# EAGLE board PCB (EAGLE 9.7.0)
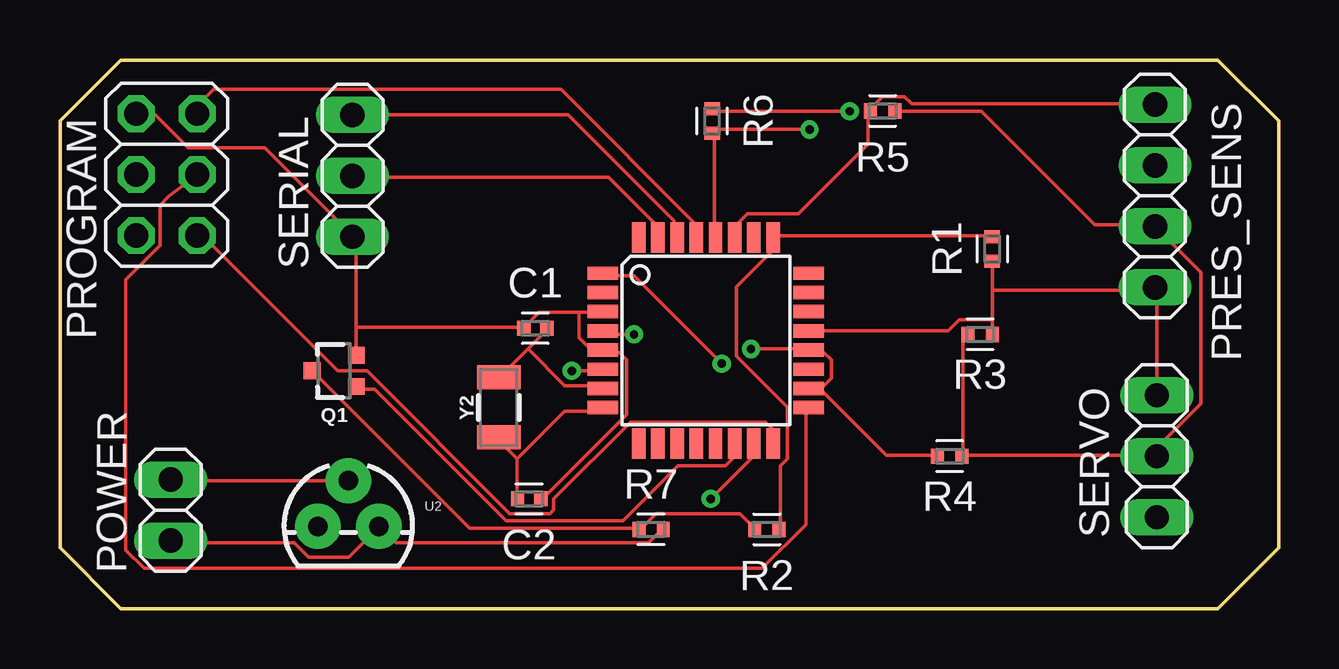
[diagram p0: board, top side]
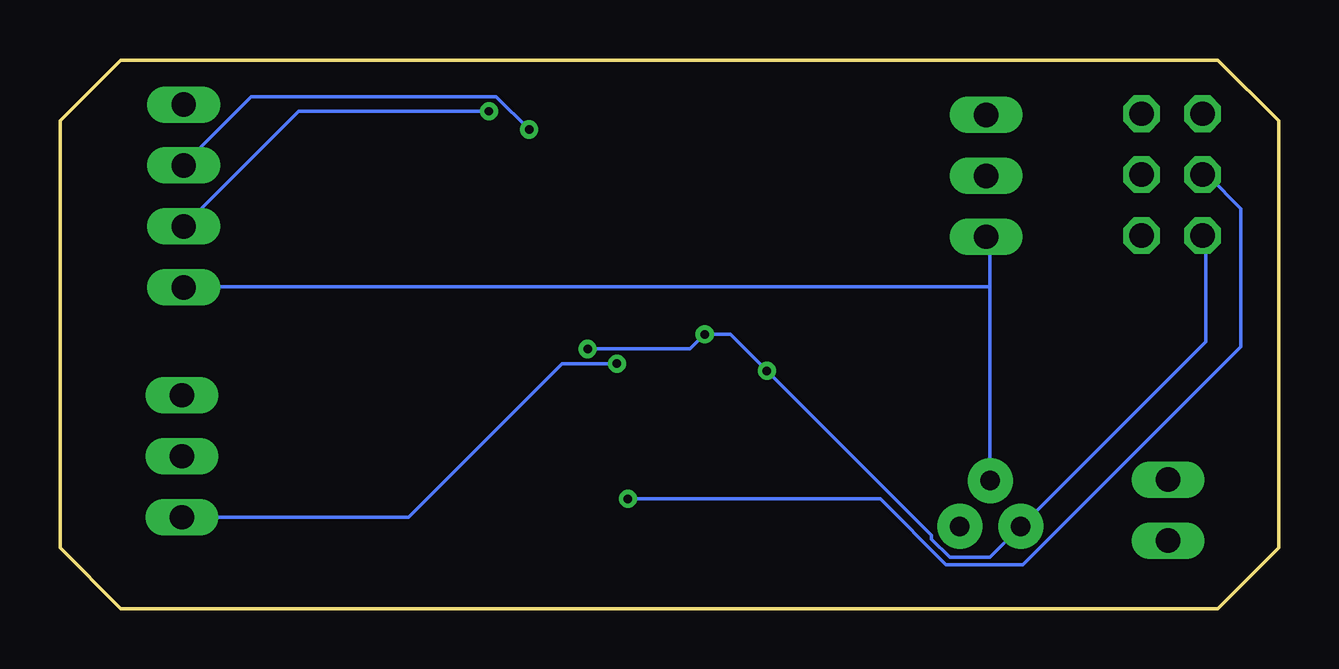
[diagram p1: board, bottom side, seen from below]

Size 50.8 x 22.86 mm. Coordinates in mm from the lower left corner, seen from the top.
Outline: 0,2.54 0,20.32 2.54,22.86 48.26,22.86 50.8,20.32 50.8,2.54 48.26,0 2.54,0 0,2.54
Copper layers (1*16): Top 0.035mm / dielectric 1.5mm / Bottom 0.035mm
Design rules "default": minimum track width 6mil, minimum drill 0.35mm, track to track 6mil, track to pad 6mil, pad to pad 6mil, via to via 6mil, smd to smd 6mil, copper to edge 40mil, drill to drill 6mil, minimum pad ring 10mil, minimum via ring 8mil, stop-mask expansion 4mil, vias tented up to drill 0mil, thermal gap 10mil

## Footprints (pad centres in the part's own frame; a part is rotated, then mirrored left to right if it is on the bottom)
CAPC1005X60 = smd 0.56 x 0.629: 1 -0.485,0; 2 0.485,0
TQFP32-08 = smd 1.27 x 0.559: 1 -4.293,2.8; 2 -4.293,2; 3 -4.293,1.2; 4 -4.293,0.4; 5 -4.293,-0.4; 6 -4.293,-1.2; 7 -4.293,-2; 8 -4.293,-2.8; 17 4.293,-2.8; 18 4.293,-2; 19 4.293,-1.2; 20 4.293,-0.4; 21 4.293,0.4; 22 4.293,1.2; 23 4.293,2; 24 4.293,2.8 | smd 0.559 x 1.27: 9 -2.8,-4.293; 10 -2,-4.293; 11 -1.2,-4.293; 12 -0.4,-4.293; 13 0.4,-4.293; 14 1.2,-4.293; 15 2,-4.293; 16 2.8,-4.293; 25 2.8,4.293; 26 2,4.293; 27 1.2,4.293; 28 0.4,4.293; 29 -0.4,4.293; 30 -1.2,4.293; 31 -2,4.293; 32 -2.8,4.293
1X02 = drill 1.016 long: 1 -1.27,0; 2 1.27,0
1X04 = drill 1.016 long: 1 -3.81,0; 2 -1.27,0; 3 1.27,0; 4 3.81,0
2X03 = drill 1.016 octagon: 1 -2.54,-1.27; 2 -2.54,1.27; 3 0,-1.27; 4 0,1.27; 5 2.54,-1.27; 6 2.54,1.27
SOT323 = smd 0.7 x 0.7: 1 -0.65,-0.925; 2 0.65,-0.925; 3 0,0.925
RESC1005X40 = smd 0.535 x 0.644: 1 -0.507,0; 2 0.507,0
1X03 = drill 1.016 long: 1 -2.54,0; 2 0,0; 3 2.54,0
TO-92 = drill 0.813 pad 1.88: 1 -1.27,0; 2 0,1.905; 3 1.27,0
CRYSTAL-SMD-3.2X1.5MM = smd 1 x 1.8: P$1 -1.25,0; P$2 1.25,0

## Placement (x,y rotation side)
C1  22p  [CAPC1005X60]  19.81,11.68 0 top
C2  22p  [CAPC1005X60]  19.56,4.57 180 top
IC1  ATMEGA328P  [TQFP32-08]  26.92,11.18 0 top
POWER  PINHD-1X2  [1X02]  4.61,4.11 90 top
PRES_SENS  PINHD-1X4  [1X04]  45.64,17.2 270 top
PROGRAM  PINHD-2X3  [2X03]  4.45,18.08 90 top
Q1  310mA/60V/1.6Ω  [SOT323]  11.43,9.91 90 top
R1  10K  [RESC1005X40]  38.86,14.99 90 top
R2  5K  [RESC1005X40]  29.46,3.3 180 top
R3  5K  [RESC1005X40]  38.35,11.43 0 top
R4  5K  [RESC1005X40]  37.08,6.35 0 top
R5  5K  [RESC1005X40]  34.29,20.74 180 top
R6  5K  [RESC1005X40]  27.18,20.32 270 top
R7  10K  [RESC1005X40]  24.64,3.3 0 top
SERIAL  PINHD-1X3  [1X03]  12.19,18.03 90 top
SERVO  PINHD-1X3  [1X03]  45.72,6.35 270 top
U2  7805  [TO-92]  12.02,3.43 0 top
Y2  16M  [CRYSTAL-SMD-3.2X1.5MM]  18.29,8.38 90 top

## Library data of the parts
C1 C2 = Capacitor; CATEGORY: Capacitor
IC1 = IC_Embedded; CATEGORY: IC_Embedded; MANUFACTURER: Microchip; MPN: ATmega328P-MMH; OPERATING_TEMP: -40 to 85 °C; PART_STATUS: Active; SUB-CATEGORY: Microcontroller
POWER PRES_SENS PROGRAM SERIAL SERVO = Connector; CATEGORY: CONNECTOR; SUB-CATEGORY: PIN-HEADER
Q1 = SparkFun-DiscreteSemi; PROD_ID: TRANS-11151
R1-R7 = Resistor; CATEGORY: Resistor; SUB-CATEGORY: Fixed
U2 = SparkFun-IC-Power
Y2 = SparkFun-Clocks

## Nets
+V: POWER.1 R7.2 U2.3
GND: C1.1 C2.1 IC1.3 IC1.5 IC1.21 POWER.2 PRES_SENS.4 PROGRAM.6 Q1.2 R1.1 R3.2 SERIAL.1 SERVO.1 U2.2
N$1: IC1.4 IC1.6 IC1.18 IC1.20 PROGRAM.2 R4.1 U2.1
N$2: C1.2 IC1.7 Y2.P$2
N$3: C2.2 IC1.8 Y2.P$1
N$4: IC1.28 PRES_SENS.2 R6.2
N$5: IC1.27 PRES_SENS.1 R5.2
N$7: IC1.14 Q1.1
N$8: IC1.25 R1.2 R2.1
N$9: Q1.3 R2.2 R7.1
N$10: PRES_SENS.3 R3.1 R4.2 R5.1 R6.1 SERVO.2
N$11: IC1.16 PROGRAM.1
N$12: IC1.17 PROGRAM.3
N$13: IC1.29 PROGRAM.5
N$14: IC1.15 PROGRAM.4
N$17: IC1.1 SERVO.3
N$18: IC1.31 SERIAL.2
N$19: IC1.30 SERIAL.3

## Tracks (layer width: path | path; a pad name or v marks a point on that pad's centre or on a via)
+V
  Top 0.152: R7.2 24.99,3.2 24.54,2.74 14.02,2.74 13.41,3.35 U2.3 13.26,3.35 12.04,2.13 10.36,2.13 9.75,2.74 4.72,2.74 POWER.1
GND
  Top 0.152: R1.1 38.86,13.26 | 38.86,13.26 38.86,12.04 | 38.86,12.04 R3.2 | 38.86,12.04 37.49,12.04 37.03,11.58 31.24,11.58 IC1.21 | SERVO.1 45.72,13.26 PRES_SENS.4 45.57,13.26 38.86,13.26 | U2.2 4.72,5.33 POWER.2 | 21.64,12.34 22.55,12.34 IC1.3 | 21.64,12.34 19.96,12.34 19.36,11.73 C1.1 19.2,11.73 12.34,11.73 | C2.1 20.12,4.57 23.62,8.08 23.62,10.36 23.32,10.67 22.71,10.67 IC1.5 22.55,10.82 22.1,10.82 21.64,11.28 21.64,12.34 | 12.34,11.73 12.34,15.24 12.19,15.39 SERIAL.1 12.19,15.54 8.53,19.2 5.33,19.2 3.96,20.57 3.3,20.57 PROGRAM.6 | 12.34,11.73 12.34,10.67 Q1.2
  Bottom 0.152: 12.04,13.41 12.04,15.24 12.19,15.39 SERIAL.1 | 12.04,13.41 12.04,5.33 U2.2 | 12.04,13.41 45.57,13.41 PRES_SENS.4
N$1  (via drill 0.35)
  Top 0.152: 31.7,9.14 34.44,6.4 36.58,6.4 R4.1 | 31.7,9.14 31.24,9.14 IC1.18 31.7,9.14 | 31.7,9.14 32.16,9.6 32.16,10.36 31.85,10.67 31.24,10.67 IC1.20 31.09,10.82 v28.8,10.82 | v21.34,9.91 22.55,9.91 IC1.6 | v23.93,11.43 22.71,11.43 IC1.4
  Bottom 0.152: PROGRAM.2 3.05,15.38 3.05,11.12 10.67,3.5 U2.1 10.82,3.35 12.04,2.13 13.72,2.13 14.48,2.9 14.48,3.05 v21.34,9.91 22.86,11.43 v23.93,11.43 24.54,10.82 v28.8,10.82
N$2
  Top 0.152: 19.51,10.82 18.29,9.6 Y2.P$2 | 19.51,10.82 20.27,11.58 C1.2 | 19.51,10.82 21.03,9.3 22.55,9.3 IC1.7
N$3
  Top 0.152: 19.05,6.25 19.05,4.57 C2.2 | 19.05,6.25 18.29,7.01 Y2.P$1 | 19.05,6.25 21.03,8.23 22.55,8.23 IC1.8
N$4  (via drill 0.35)
  Top 0.152: IC1.28 27.28,15.54 27.28,19.81 R6.2 27.28,19.96 v31.24,19.96
  Bottom 0.152: v31.24,19.96 32.61,21.34 42.82,21.34 45.57,18.59 PRES_SENS.2
N$5
  Top 0.152: IC1.27 28.19,15.54 28.19,16 28.65,16.46 30.79,16.46 33.68,19.36 33.68,20.73 R5.2 33.83,20.88 34.29,21.34 35.2,21.34 35.51,21.03 45.57,21.03 PRES_SENS.1
N$7
  Top 0.152: Q1.1 12.5,9.14 13.11,9.14 18.59,3.66 23.47,3.66 25.76,5.94 27.74,5.94 28.04,6.25 28.04,6.86 IC1.14
N$8
  Top 0.152: R2.1 30.02,3.35 30.02,5.94 30.33,6.25 30.33,8.38 28.19,10.52 28.19,13.41 29.72,14.94 29.72,15.39 IC1.25 29.87,15.54 38.86,15.54 R1.2
N$9
  Top 0.152: R2.2 28.96,3.35 28.35,3.96 24.84,3.96 24.23,3.35 R7.1 24.08,3.35 17.07,3.35 10.52,9.91 Q1.3
N$10  (via drill 0.35)
  Top 0.152: 37.64,6.4 37.64,11.28 37.8,11.43 R3.1 | 45.72,6.4 37.64,6.4 | 37.64,6.4 R4.2 | v32.92,20.73 27.28,20.73 R6.1 | R5.1 34.9,20.73 38.41,20.73 43.13,16 45.57,16 PRES_SENS.3 47.55,14.02 47.55,8.53 45.72,6.71 45.72,6.4 | 45.72,6.4 SERVO.2
  Bottom 0.152: v32.92,20.73 40.84,20.73 PRES_SENS.3
N$11
  Top 0.152: IC1.16 29.72,7.01 29.72,7.47 29.41,7.77 23.77,7.77 20.57,4.57 20.57,4.12 20.42,3.96 18.75,3.96 12.8,9.91 11.58,9.91 6.1,15.39 5.74,15.39 PROGRAM.1
N$12
  Top 0.152: IC1.17 31.09,8.23 31.09,3.5 29.26,1.68 3.5,1.68 2.74,2.44 2.74,13.71 4.17,15.13 4.17,16.82 4.54,17.19 PROGRAM.3
N$13
  Top 0.152: IC1.29 26.52,15.54 26.52,16 20.88,21.64 6.4,21.64 5.81,21.05 PROGRAM.5
N$14  (via drill 0.35)
  Top 0.152: v27.13,4.57 28.8,6.25 28.8,6.86 IC1.15
  Bottom 0.152: v27.13,4.57 16.61,4.57 13.87,1.83 10.67,1.83 1.57,10.92 1.57,16.66 2.92,18.01 PROGRAM.4
N$17  (via drill 0.35)
  Top 0.152: v27.58,10.21 23.93,13.87 22.71,13.87 IC1.1
  Bottom 0.152: v27.58,10.21 29.87,10.21 36.27,3.81 SERVO.3
N$18
  Top 0.152: IC1.31 24.84,15.54 24.84,16 22.86,17.98 12.19,17.98 SERIAL.2
N$19
  Top 0.152: SERIAL.3 21.18,20.57 25.6,16.15 25.6,15.54 IC1.30

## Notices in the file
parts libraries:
SparkFun-DiscreteSemi: Licensing: Creative Commons ShareAlike 4.0 International - https://creativecommons.org/licenses/by-sa/4.0
